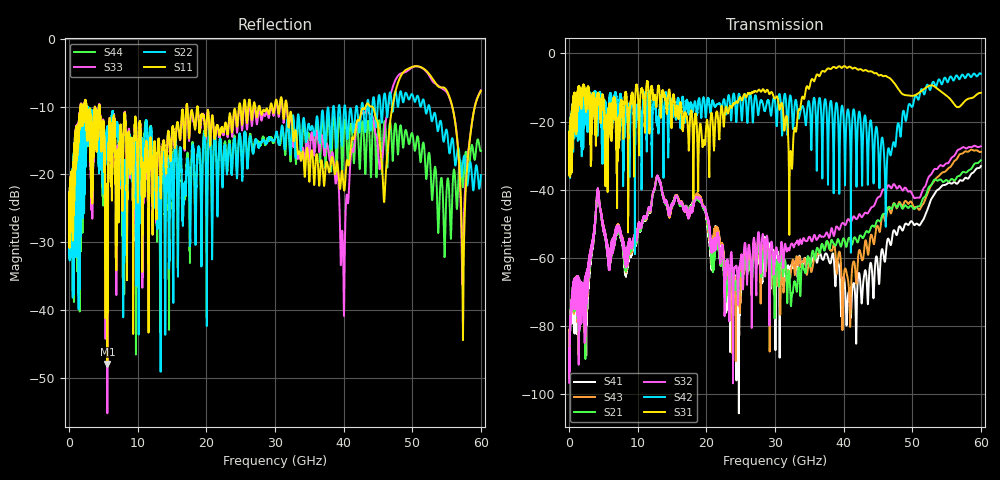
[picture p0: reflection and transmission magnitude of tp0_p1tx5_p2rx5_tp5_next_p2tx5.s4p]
! 100G CR Analysis
! File: tp0_p1tx5_p2rx5_tp5_next_p2tx5
! Description: 2m Cu Cable, OSFP, TP0-TP5
! Port Mapping
! Port1 -- P2TX5N
! Port2 -- P2RX5N
! Port3 -- P2TX5P
! Port4 -- P2RX5P
# GHz S MA R 50.00
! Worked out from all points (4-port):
!   6000 points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, 10 MHz to 60 GHz, reference 50 ohm
!   strongest paths, dB at 10 MHz, 15.01 GHz, 30.01 GHz, 45.01 GHz, 60 GHz:
!     S31: -28.0, -16.7, -13.2, -6.3, -11.6
!     S42: -27.9, -17.3, -14.1, -26.1, -6.0
!     S32: -96.7, -44.1, -59.4, -42.3, -27.3
!     S21: -95.3, -44.2, -71.0, -49.0, -31.4
!     S43: -91.9, -44.3, -64.3, -50.9, -28.9
!     S41: -91.0, -44.2, -68.5, -63.3, -33.1
!   lowest |S11| = -47.9 dB at 5.58 GHz (marker M1), VSWR 1.01, Z = 50.4 + j0.0868 ohm
!   |S11| at or under -10 dB: 4.457 GHz to 17.09 GHz (12.63 GHz wide, 117 % of centre); 18.71 GHz to 24.75 GHz (6.034 GHz wide, 27.8 % of centre); 31.75 GHz to 43.21 GHz (11.46 GHz wide, 30.6 % of centre)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
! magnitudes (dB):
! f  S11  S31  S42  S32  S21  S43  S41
! 10 MHz  -23.8  -28.0  -27.9  -96.7  -95.3  -91.9  -91.0
! 5.58 GHz  -47.9  -22.1  -20.2  -57.6  -57.9  -57.7  -58.0
! 12.96 GHz  -15.6  -9.9  -20.3  -36.2  -36.4  -36.3  -36.4
! 24.62 GHz  -11.6  -14.3  -13.0  -72.3  -71.5  -69.9  -73.3
! 32.29 GHz  -10.8  -28.7  -12.6  -56.3  -73.3  -65.1  -62.8
! 40.86 GHz  -18.0  -3.9  -20.1  -49.0  -54.3  -73.0  -71.6
! 60 GHz  -7.7  -11.6  -6.0  -27.3  -31.4  -28.9  -33.1
